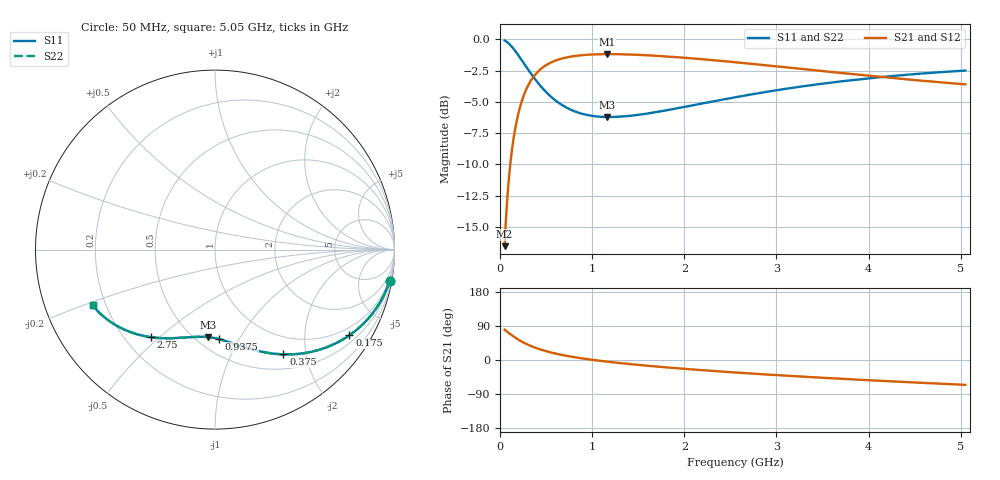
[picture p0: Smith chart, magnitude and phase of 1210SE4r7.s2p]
! AVX Thin Film Operation		Date: August 2001
! Description: Accu-P® Series, Thin Film, SMD, RF Capacitor
! Part Number: 12101J4R7ABT
! 50 MHz  -  5.05 GHz
! Serial Measurements
# mhz S db R 50
!	S11		S21		S12		S22
!	dB	Phase	dB	Phase	dB	Phase	dB	Phase
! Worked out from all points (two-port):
!   401 points, 50 MHz to 5.05 GHz, reference 50 ohm
!   highest |S21| = -1.19 dB at 1.163 GHz (marker M1); lowest = -16.5 dB at 50 MHz (marker M2)
!   |S21| within 3 dB of the highest: 273.7 MHz to end of sweep
!   lowest |S11| = -6.2 dB at 1.163 GHz (marker M3), VSWR 2.91, Z = 29 - j37.1 ohm
!   |S11| at or under -10 dB: nowhere
!   |S22| runs from -6.2 to -0.1 dB; largest |S21 - S12| = 0
!   S11 on the Smith chart (normalised r, x): 50 MHz: 1, -11; 175 MHz: 0.73, -3.28; 375 MHz: 0.71, -1.61; 937.5 MHz: 0.62, -0.83; 2.75 GHz: 0.31, -0.47; 5.05 GHz: 0.15, -0.21
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50  -0.10 -10.1  -16.53 79.9  -16.53 79.9  -0.10 -10.1
75  -0.22 -14.9  -13.14 75.1  -13.14 75.1  -0.22 -14.9
112.5  -0.47 -21.9  -9.92 68.1  -9.92 68.1  -0.47 -21.9
137.5  -0.68 -26.4  -8.42 63.6  -8.42 63.6  -0.68 -26.4
175  -1.03 -32.5  -6.75 57.5  -6.75 57.5  -1.03 -32.5
212.5  -1.42 -38.2  -5.55 51.8  -5.55 51.8  -1.42 -38.2
262.5  -1.96 -44.8  -4.39 45.2  -4.39 45.2  -1.96 -44.8
375  -3.14 -56.9  -2.89 33.1  -2.89 33.1  -3.14 -56.9
475  -4.02 -65.0  -2.19 25.0  -2.19 25.0  -4.02 -65.0
587.5  -4.80 -72.1  -1.75 17.8  -1.75 17.8  -4.80 -72.2
725  -5.48 -79.1  -1.45 10.9  -1.45 10.9  -5.48 -79.1
887.5  -5.95 -85.6  -1.28 4.4  -1.28 4.4  -5.95 -85.6
937.5  -6.04 -87.4  -1.25 2.6  -1.25 2.6  -6.04 -87.4
1162.5  -6.21 -94.3  -1.19 -4.4  -1.19 -4.4  -6.21 -94.4
1425  -6.11 -101.1  -1.22 -11.2  -1.22 -11.2  -6.11 -101.2
1725  -5.78 -107.8  -1.34 -17.8  -1.34 -17.8  -5.78 -107.8
2125  -5.23 -115.6  -1.55 -25.6  -1.55 -25.6  -5.23 -115.6
2550  -4.64 -122.9  -1.83 -32.9  -1.83 -32.9  -4.64 -122.9
2750  -4.38 -126.1  -1.98 -36.1  -1.98 -36.1  -4.38 -126.1
3387.5  -3.66 -135.4  -2.46 -45.4  -2.46 -45.4  -3.66 -135.4
4225  -2.96 -146.1  -3.08 -56.1  -3.08 -56.1  -2.96 -146.1
5050  -2.50 -155.5  -3.60 -65.6  -3.60 -65.6  -2.50 -155.5
